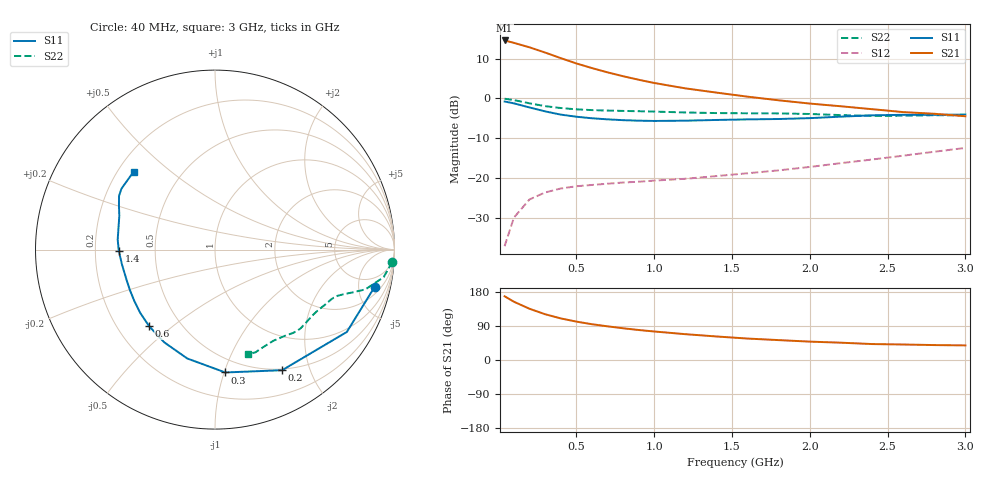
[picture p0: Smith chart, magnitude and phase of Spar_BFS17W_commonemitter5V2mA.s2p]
! Filename:  BFS17WA.S2P  Version:  4.0
! NXP part #: BFS17W  Date: Jun 1994
! Bias condition: Vce=5V, Ic=2mA
#  MHz  S  MA  R  50
! Freq  S11  S21  S12  S22  !GUM [dB]
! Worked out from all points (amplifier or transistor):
!   21 points, 40 MHz to 3 GHz, reference 50 ohm
!   highest |S21| = 14.5 dB at 40 MHz (marker M1)
!   |S21| within 3 dB of that: start of sweep to 297.7 MHz
!   unconditionally stable (mu >= 1): 807.9 MHz to end of sweep
!   at 300 MHz: K = 0.49, MSG = 17.6 dB, |S12| = -23.6 dB
!   at 1 GHz: K = 1.17, MAG = 9.8 dB, |S12| = -20.6 dB
!   at 3 GHz: K = 1.21, MAG = 1.2 dB, |S12| = -12.4 dB
!   S11 on the Smith chart (normalised r, x): 40 MHz: 2.98, -7.47; 200 MHz: 0.48, -1.59; 300 MHz: 0.39, -1.01; 600 MHz: 0.33, -0.42; 1.4 GHz: 0.30, -0.01; 3 GHz: 0.26, +0.38
40  0.913 -13.2  5.327 168.1  0.014 82.2  0.99 -4.0
100  0.866 -32.0  4.969 153.7  0.032 69.9  0.952 -9.3
200  0.769 -60.9  4.368 135.2  0.054 56.6  0.867 -14.8
300  0.687 -85.2  3.758 120.8  0.066 48.8  0.8 -17.4
400  0.626 -104.3  3.201 109.8  0.074 45.0  0.757 -19.2
500  0.589 -118.7  2.746 101.4  0.079 43.6  0.729 -20.7
600  0.563 -130.6  2.402 94.5  0.082 43.5  0.713 -22.1
700  0.546 -139.7  2.122 88.9  0.085 44.4  0.703 -23.4
800  0.533 -147.5  1.898 83.8  0.088 45.9  0.696 -24.6
900  0.525 -154.5  1.715 79.2  0.09 47.6  0.69 -25.8
1000  0.521 -160.5  1.561 75.3  0.093 49.8  0.683 -27.1
1200  0.525 -171.0  1.336 68.2  0.098 54.3  0.666 -30.4
1400  0.536 -179.2  1.182 62.1  0.106 59.4  0.654 -34.6
1600  0.545 174.1  1.051 56.6  0.115 64.3  0.65 -39.1
1800  0.551 167.4  0.946 52.5  0.125 69.4  0.648 -42.9
2000  0.565 160.7  0.861 48.5  0.138 73.9  0.637 -46.7
2200  0.59 155.1  0.796 45.7  0.154 77.8  0.617 -51.4
2400  0.613 150.7  0.732 42.1  0.171 80.7  0.603 -57.5
2600  0.622 146.9  0.673 40.9  0.191 82.6  0.606 -63.7
2800  0.622 142.1  0.641 39.4  0.214 84.3  0.615 -68.5
3000  0.627 136.4  0.597 38.5  0.239 85.4  0.612 -72.3
